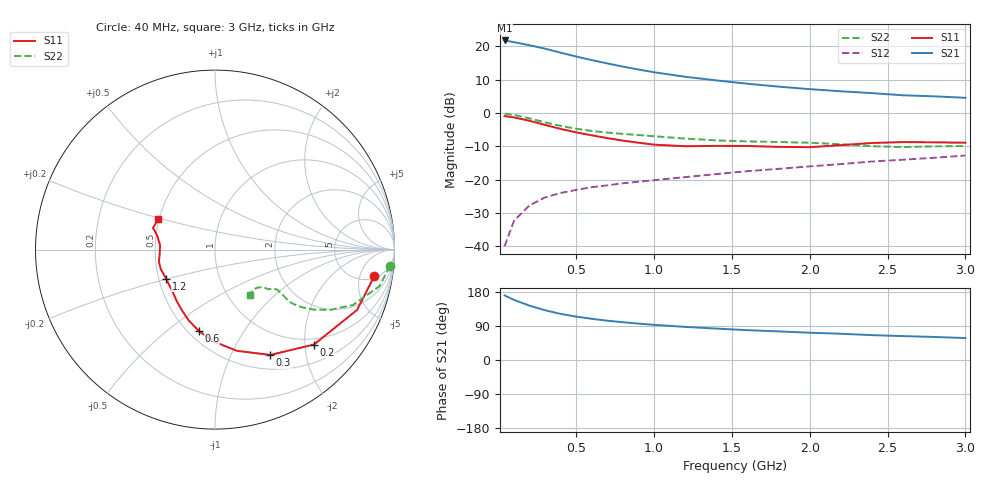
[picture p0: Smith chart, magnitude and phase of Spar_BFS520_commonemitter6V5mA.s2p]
! Filename:  BFS520H.S2P  Version:  4.0
! NXP part #: BFS520  Date: Jun 1994
! Bias condition: Vce=6V, Ic=5mA
#  MHz  S  MA  R  50
! Freq  S11  S21  S12  S22  !GUM [dB]
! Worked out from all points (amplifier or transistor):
!   21 points, 40 MHz to 3 GHz, reference 50 ohm
!   highest |S21| = 21.8 dB at 40 MHz (marker M1)
!   |S21| within 3 dB of that: start of sweep to 343.9 MHz
!   unconditionally stable (mu >= 1): 1.068 GHz to end of sweep
!   at 300 MHz: K = 0.43, MSG = 22.3 dB, |S12| = -25.4 dB
!   at 1 GHz: K = 0.97, MSG = 16.2 dB, |S12| = -20.2 dB
!   at 3 GHz: K = 1.10, MAG = 6.8 dB, |S12| = -12.8 dB
!   lowest NFmin = 0.90 dB at 500 MHz
!   S11 on the Smith chart (normalised r, x): 40 MHz: 6, -9; 200 MHz: 0.87, -2.20; 300 MHz: 0.68, -1.43; 600 MHz: 0.56, -0.65; 1.2 GHz: 0.55, -0.20; 3 GHz: 0.50, +0.19
40  0.9 -9.4  12.31 170.3  0.01 84.3  0.98 -5.3
100  0.86 -23.0  11.61 158.7  0.024 75.8  0.938 -12.6
200  0.764 -43.8  10.44 143.4  0.041 65.3  0.828 -21.9
300  0.663 -62.3  9.258 131.3  0.054 59.4  0.723 -27.7
400  0.577 -77.8  8.062 121.7  0.063 56.4  0.641 -31.4
500  0.513 -90.6  7.058 114.5  0.07 54.9  0.58 -33.6
600  0.462 -101.3  6.235 108.7  0.077 54.9  0.538 -34.6
700  0.42 -110.6  5.554 103.7  0.082 55.5  0.508 -35.0
800  0.385 -118.6  4.976 99.7  0.088 56.3  0.486 -34.6
900  0.358 -126.5  4.503 96.0  0.093 57.2  0.467 -34.1
1000  0.335 -134.3  4.098 92.8  0.098 58.2  0.448 -33.5
1200  0.317 -149.3  3.504 87.4  0.109 60.3  0.413 -32.8
1400  0.321 -160.2  3.093 82.9  0.121 62.3  0.388 -33.8
1600  0.32 -167.6  2.753 78.7  0.134 63.6  0.375 -36.0
1800  0.31 -174.7  2.492 75.5  0.145 65.5  0.367 -36.9
2000  0.307 175.4  2.284 72.0  0.158 66.7  0.358 -37.1
2200  0.329 167.0  2.122 69.3  0.171 67.9  0.339 -38.0
2400  0.355 162.2  1.99 65.6  0.187 68.6  0.318 -41.6
2600  0.366 160.9  1.847 63.1  0.199 68.8  0.308 -47.1
2800  0.363 158.1  1.781 60.8  0.213 69.8  0.316 -50.9
3000  0.358 152.0  1.694 57.9  0.23 70.1  0.32 -52.5
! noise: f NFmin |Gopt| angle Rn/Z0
500  0.9  0.359  27  0.24
900  1.1  0.338  45  0.23
2000  1.85  0.277  161  0.13
